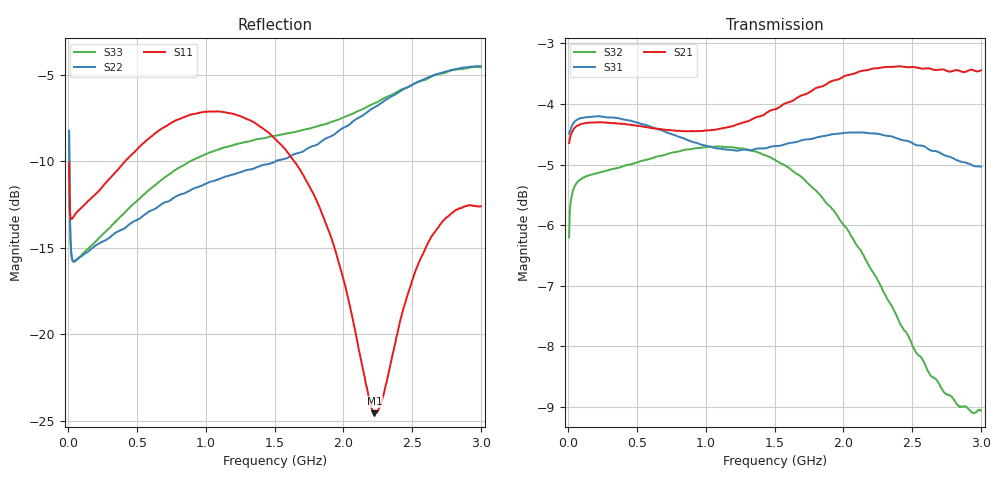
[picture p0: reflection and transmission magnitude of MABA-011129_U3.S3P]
!Agilent Technologies,E5071C,MY46630996,B.13.30
!Date: Tue Aug 16 22:18:44 2022 DD
!Data & Calibration Information:
!MABA-011129-TB soldered onto PT-0028476 with SMA connectors, Port1 (pin1) Port2 (pin4) Port3 (pin3)
!Freq	S11:SOLT3(ON)	S12:SOLT3(ON)	S13:SOLT3(ON)
!	S21:SOLT3(ON)	S22:SOLT3(ON)	S23:SOLT3(ON)
!	S31:SOLT3(ON)	S32:SOLT3(ON)	S33:SOLT3(ON)
!PortZ  Port1:50+j0  Port2:50+j0  Port3:50+j0
!Above PortZ is port z conversion or system Z0 setting when saving the data.
!When reading, reference impedance value at option line is always used.
# Hz S dB R 50
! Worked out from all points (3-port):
!   600 points, 5 MHz to 3 GHz, reference 50 ohm
!   strongest paths, dB at 5 MHz, 755 MHz, 1.505 GHz, 2.255 GHz, 3 GHz:
!     S21: -4.6, -4.4, -4.1, -3.4, -3.4
!     S31: -4.5, -4.5, -4.7, -4.5, -5.0
!     S32: -6.2, -4.8, -4.9, -6.9, -9.1
!   lowest |S11| = -24.6 dB at 2.225 GHz (marker M1), VSWR 1.13, Z = 44.4 - j0.0171 ohm
!   |S11| at or under -10 dB: start of sweep to 411.6 MHz; 1.643 GHz to end of sweep
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5000000  -10.07 60.9  -4.71 -166.6  -4.53 12.8
         -4.64 -166.6  -8.22 91.0  -6.18 30.2
         -4.49 12.7  -6.20 30.1  -8.32 89.6
2.5e7  -13.33 14.5  -4.47 -178.7  -4.36 1.1
       -4.47 -178.7  -15.58 37.5  -5.50 6.3
       -4.36 1.1  -5.51 6.3  -15.61 35.3
4.5e7  -13.11 3.3  -4.40 178.3  -4.29 -1.7
       -4.39 178.3  -15.75 21.3  -5.35 2.8
       -4.29 -1.7  -5.36 2.8  -15.80 18.2
6.15e8  -8.48 -102.9  -4.42 126.8  -4.32 -53.5
        -4.40 126.7  -12.80 -57.4  -4.90 -27.7
        -4.39 -53.6  -4.89 -27.8  -11.47 -72.5
1.085e9  -7.10 -153.6  -4.41 87.9  -4.58 -93.4
         -4.42 87.7  -11.03 -85.8  -4.71 -52.6
         -4.74 -92.7  -4.70 -53.0  -9.33 -102.6
1.505e9  -8.71 169.4  -4.10 53.3  -4.67 -128.2
         -4.08 53.0  -10.00 -99.2  -4.94 -77.0
         -4.69 -127.0  -4.93 -77.7  -8.51 -118.6
1.905e9  -14.27 141.8  -3.67 18.4  -4.57 -162.5
         -3.63 18.0  -8.56 -106.5  -5.68 -101.0
         -4.50 -161.9  -5.69 -101.6  -7.74 -129.1
2.225e9  -24.58 -179.8  -3.47 -11.0  -4.57 168.3
         -3.41 -11.3  -6.87 -114.9  -6.81 -119.1
         -4.49 168.4  -6.81 -119.4  -6.64 -137.1
2.625e9  -14.57 -137.4  -3.46 -47.8  -4.78 131.1
         -3.41 -48.0  -5.11 -130.2  -8.54 -136.4
         -4.76 130.7  -8.45 -136.1  -5.16 -150.4
3e9  -12.59 -158.2  -3.52 -81.5  -5.03 96.3
     -3.44 -81.1  -4.48 -145.2  -9.29 -147.4
     -5.03 96.1  -9.06 -147.0  -4.54 -162.7
